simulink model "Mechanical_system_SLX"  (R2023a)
settings: Solver=ode23s  StartTime=0.0  StopTime=10.0  MaxStep=0.001  RelTol=1e-3
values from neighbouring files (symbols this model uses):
  b_3 = 0.1*Nm/(rad/sec)    (= 0.1)    [Mechanical_system_EQN.m]    (also in Mechanical_system_SLX_m.m; Car_Dumper_EQN.m = 2; Car_Dumper_SLX_m.m = 2; Mechanical_Mass_Spring_Mass_EQN.m = 2)
  b_8 = 2*N/(m/sec)    (= 2)    [Mechanical_system_EQN.m]    (also in Mechanical_system_SLX_m.m)
  F_6_0 = 0*N    (= 0)    [Mechanical_system_SLX_m.m]
  F_9_0 = 0*N    (= 0)    [Mechanical_system_SLX_m.m]
  J_2 = 0.01*kg*m^2    (= 0.01)    [Mechanical_system_EQN.m]    (also in Mechanical_system_SLX_m.m; Rotational_Inertias_and_Dumper_EQN.m; Rotational_Inertias_and_Dumper_SLX_m.m)
  K_6 = 1000*N/m    (= 1000)    [Mechanical_system_EQN.m]    (also in Mechanical_system_SLX_m.m)
  K_9 = 1000*N/m    (= 1000)    [Mechanical_system_EQN.m]    (also in Mechanical_system_SLX_m.m)
  M_7 = 0.5*kg    (= 0.5)    [Mechanical_system_EQN.m]    (also in Mechanical_system_SLX_m.m)
  R = 1    [Mechanical_system_EQN.m]    (also in Mechanical_system_SLX_m.m; Electrical_Transformer_EQN.m; Electrical_Transformer_SLX_m.m; Mechanical_Transmission_EQN.m)
  T_1_0 = 10*Nm    (= 10)    [Mechanical_system_SLX_m.m]    (also in Rotational_Inertias_and_Dumper_SLX_m.m)
  Ts = Tfin/Nr_Ts_Points    (= 0.0014555)    [Mechanical_system_SLX_m.m]    (also in BIG_EC_Simscape_SLX_m.m = 0.0003; Car_Dumper_SLX_m.m = 0.0022779; Electric_Circuit_01_SLX_m.m = 0.005; Electric_Circuit_02_SLX_m.m = 0.000480145)
  v_7_0 = 0*m/sec    (= 0)    [Mechanical_system_SLX_m.m]
  v_b_0 = 0*m/sec    (= 0)    [Mechanical_system_SLX_m.m]
  w_2_0 = 0*rad/sec    (= 0)    [Mechanical_system_SLX_m.m]    (also in Rotational_Inertias_and_Dumper_SLX_m.m)

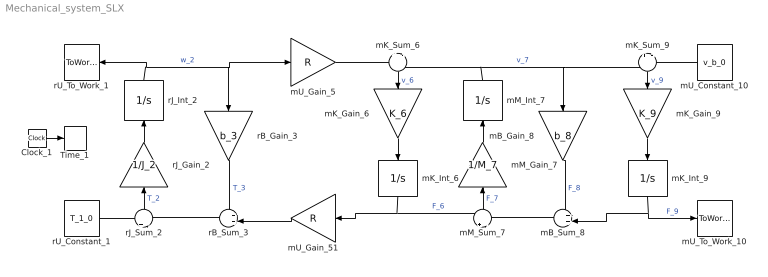
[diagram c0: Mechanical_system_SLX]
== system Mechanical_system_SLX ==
  Clock_1 : Clock
  Time_1 : ToWorkspace  VariableName=t  SaveFormat=Timeseries  SampleTime=Ts
  mB_Gain_8 : Gain  Gain=b_8  Multiplication=Matrix(K*u)
  mB_Sum_8 : Sum  Inputs=++|
  mK_Gain_6 : Gain  Gain=K_6  Multiplication=Matrix(K*u)
  mK_Gain_9 : Gain  Gain=K_9  Multiplication=Matrix(K*u)
  mK_Int_6 : Integrator  InitialCondition=F_6_0
  mK_Int_9 : Integrator  InitialCondition=F_9_0
  mK_Sum_6 : Sum  Inputs=+|-
  mK_Sum_9 : Sum  Inputs=+|-
  mM_Gain_7 : Gain  Gain=1/M_7  Multiplication=Matrix(K*u)
  mM_Int_7 : Integrator  InitialCondition=v_7_0
  mM_Sum_7 : Sum  Inputs=+|-
  mU_Constant_10 : Constant  Value=v_b_0
  mU_Gain_5 : Gain  Gain=R  Multiplication=Matrix(K*u)
  mU_Gain_51 : Gain  Gain=R  Multiplication=Matrix(K*u)
  mU_To_Work_10 : ToWorkspace  VariableName=F_b_0  SaveFormat=Timeseries  SampleTime=Ts
  rB_Gain_3 : Gain  Gain=b_3  Multiplication=Matrix(K*u)
  rB_Sum_3 : Sum  Inputs=++|
  rJ_Gain_2 : Gain  Gain=1/J_2  Multiplication=Matrix(K*u)
  rJ_Int_2 : Integrator  InitialCondition=w_2_0
  rJ_Sum_2 : Sum  Inputs=+|-
  rU_Constant_1 : Constant  Value=T_1_0
  rU_To_Work_1 : ToWorkspace  VariableName=w_1_0  SaveFormat=Timeseries  SampleTime=Ts
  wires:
  rU_Constant_1/1 -> rJ_Sum_2/1
  rB_Sum_3/1 -> rJ_Sum_2/2
  rJ_Int_2/1 -> rU_To_Work_1/1, rB_Gain_3/1, mU_Gain_5/1  "w_2"
  rJ_Sum_2/1 -> rJ_Gain_2/1  "T_2"
  rJ_Gain_2/1 -> rJ_Int_2/1
  mU_Gain_51/1 -> rB_Sum_3/2
  rB_Gain_3/1 -> rB_Sum_3/1  "T_3"
  mU_Gain_5/1 -> mK_Sum_6/1
  mK_Int_6/1 -> mU_Gain_51/1, mM_Sum_7/1  "F_6"
  mM_Int_7/1 -> mK_Sum_6/2, mB_Gain_8/1, mK_Sum_9/1  "v_7"
  mK_Sum_6/1 -> mK_Gain_6/1  "v_6"
  mK_Gain_6/1 -> mK_Int_6/1
  mB_Sum_8/1 -> mM_Sum_7/2
  mM_Sum_7/1 -> mM_Gain_7/1  "F_7"
  mM_Gain_7/1 -> mM_Int_7/1
  mK_Int_9/1 -> mB_Sum_8/2, mU_To_Work_10/1  "F_9"
  mB_Gain_8/1 -> mB_Sum_8/1  "F_8"
  mU_Constant_10/1 -> mK_Sum_9/2
  mK_Sum_9/1 -> mK_Gain_9/1  "v_9"
  mK_Gain_9/1 -> mK_Int_9/1
  Clock_1/1 -> Time_1/1
